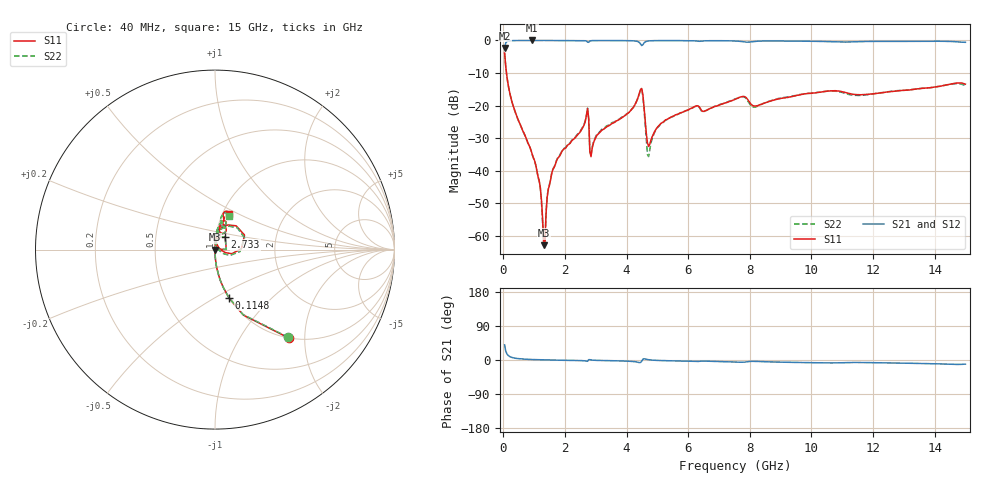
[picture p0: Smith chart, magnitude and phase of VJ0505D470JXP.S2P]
! VJ0505D470JXP
! MLCC placed on 25 mil thick microstrip substrate in series configuraton.
! DATE 06/29/2018  09:20
! CORRECTED  DATA
# GHz  S  MA  R  50.00
!  FREQ  S11M  S11A  S21M  S21A  S12M  S12A  S22M  S22A
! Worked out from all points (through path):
!   401 points, 40 MHz to 15 GHz, reference 50 ohm
!   highest |S21| = -0.02 dB at 937.6 MHz (marker M1); lowest = -2.3 dB at 40 MHz (marker M2)
!   group delay of S21, straight-line fit = 2.56 ps
!   lowest |S11| = -62.9 dB at 1.312 GHz (marker M3), VSWR 1.00, Z = 50 - j0.0667 ohm
!   |S11| at or under -10 dB: 101.5 MHz to end of sweep
!   |S22| runs from -63.1 to -3.9 dB; largest |S21 - S12| = 0.0026
!   S11 on the Smith chart (normalised r, x): 40 MHz: 1.00, -1.68; 114.8 MHz: 1.00, -0.58; 2.733 GHz: 1.11, +0.16; 15 GHz: 1.07, +0.45
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0.04  0.643 -50.1  0.7665 39.9  0.7671 39.9  0.6374 -50.1
0.1148  0.2786 -74.0  0.9588 16.2  0.9599 16.2  0.2763 -74.1
0.3392  0.0924 -85.1  0.9943 5.3  0.9946 5.4  0.09156 -85.3
0.9376  0.01788 -88.7  0.9982 1.3  0.9984 1.4  0.01752 -90.2
1.1246  0.00824 -88.1  0.998 0.8  0.9981 0.9  0.00807 -93.6
1.3116  0.0007191 -68.0  0.9976 0.4  0.9979 0.5  0.0006992 -131.0
1.3864  0.00227 73.6  0.9975 0.3  0.9978 0.3  0.002376 91.8
1.4986  0.006096 83.1  0.9971 0.1  0.9978 0.1  0.006239 91.7
1.6482  0.01129 85.3  0.9976 -0.2  0.9976 -0.1  0.01145 89.9
2.5458  0.04336 84.9  0.994 -1.7  0.9941 -1.6  0.04446 85.3
2.7328  0.09032 51.4  0.9427 -3.3  0.9434 -3.3  0.0915 51.8
2.8824  0.02213 76.9  0.9924 -0.3  0.9926 -0.2  0.02309 78.1
3.1068  0.03773 85.9  0.9953 -1.2  0.9955 -1.1  0.03875 86.8
4.4532  0.1774 48.4  0.8831 -6.6  0.8835 -6.6  0.1737 44.1
4.528  0.1478 1.9  0.8552 1.9  0.8555 1.9  0.1396 -4.5
4.715  0.0237 33.6  0.9818 0.7  0.9823 0.8  0.01653 42.7
5.0516  0.04946 82.1  0.9928 -1.3  0.9935 -1.2  0.04837 87.5
7.52  0.1252 79.5  0.9796 -5.4  0.9802 -5.3  0.1264 80.5
8.1558  0.09866 68.4  0.9661 -3.6  0.9666 -3.5  0.09489 72.4
10.0258  0.1555 76.5  0.9678 -7.1  0.9693 -7.1  0.1561 76.3
12.5316  0.1632 74.0  0.9672 -7.8  0.9677 -7.9  0.1642 77.6
15  0.2133 68.5  0.9355 -10.8  0.9363 -10.9  0.2019 66.8
